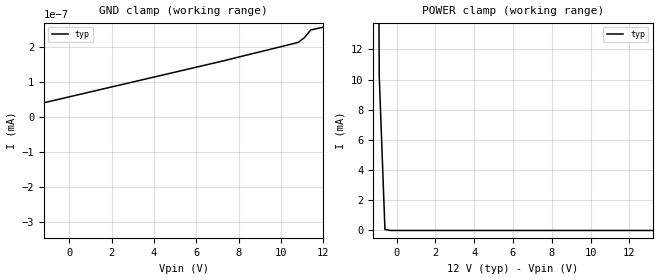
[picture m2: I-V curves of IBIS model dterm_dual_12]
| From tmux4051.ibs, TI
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| dterm_dual_12
[Model]   dterm_dual_12
Model_type   Terminator
|   typ   min   max
C_comp   6.362683e-12   NA   NA
[Voltage Range]   12   NA   NA
[Temperature Range]   27   NA   NA
[Power Clamp Reference]   12   NA   NA
[GND Clamp Reference]   0   NA   NA
[GND Clamp]
|   Voltage   I(typ)   I(min)   I(max)
-17V      -3.643A    NA         NA
-12.61V   -5.768uA   NA         NA
-12.31V   -173.1pA   NA         NA
-12.02V   -138.3pA   NA         NA
-11.43V   -129.5pA   NA         NA
-11.14V   -116.7pA   NA         NA
-10.85V   -97.64pA   NA         NA
7.313V    161.2pA    NA         NA
10.83V    213.7pA    NA         NA
11.12V    227.6pA    NA         NA
11.41V    249pA      NA         NA
12V       256.8pA    NA         NA
[POWER Clamp]
|   Voltage   I(typ)   I(min)   I(max)
-5V       2.031A     NA         NA
-1.192V   78.03mA    NA         NA
-899mV    10.19mA    NA         NA
-606.1mV  63.2uA     NA         NA
-313.1mV  12.07nA    NA         NA
24V       -138pA     NA         NA
